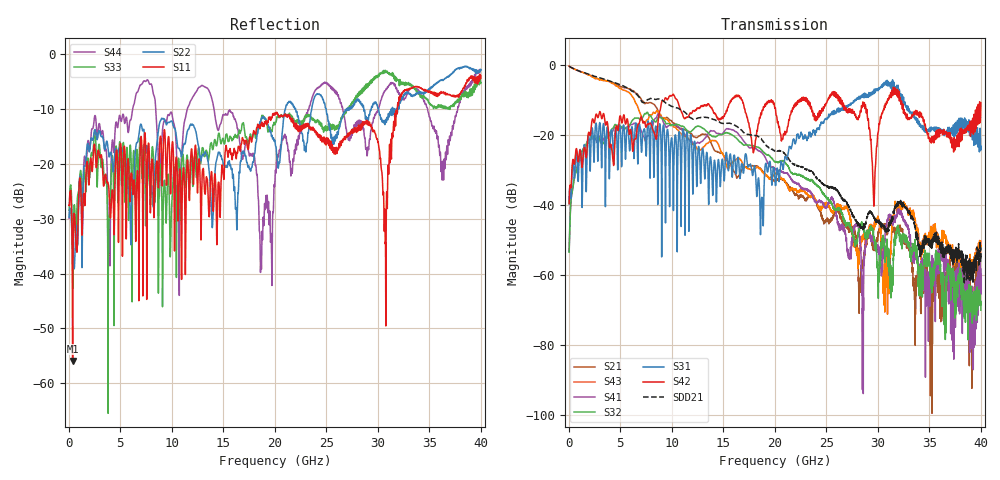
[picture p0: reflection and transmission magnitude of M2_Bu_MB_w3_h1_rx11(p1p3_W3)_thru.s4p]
! S11 = S11
! S12 = S12
! S13 = S13
! S14 = S14
! S21 = S21
! S22 = S22
! S23 = S23
! S24 = S24
! S31 = S31
! S32 = S32
! S33 = S33
! S34 = S34
! S41 = S41
! S42 = S42
! S43 = S43
! S44 = S44
! FILE: \\englab.brocade.com\shares\Groups\SIT\Work\Shaohua\IEEE_channels\M2_Bu_MB_w3_h1_rx11(p1p3_W3)_thru.s4p
!$DUT_CFG_DESC: Default 4-Port Configuration
!$NUMBER_PORTS: 4
!$DIFF_PORT_MAP: 1|2P|2|2P|0|UC|0|UC|
!$PORT_MAP: PNA 1|1|<<<<<<|TS 2|2|>>>>>>|PNA 2|3|<<<<<<|TS 4|4|>>>>>>|
# MHz S RI R 50.00
! FREQ  S11  S12  S13  S14
!  S21  S22  S23  S24
!  S31  S32  S33  S34
!  S41  S42  S43  S44
!  REAL  IMAG  REAL  IMAG  REAL  IMAG  REAL  IMAG
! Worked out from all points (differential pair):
!   3996 points, 50 MHz to 40 GHz, reference 50 ohm
!   strongest paths, dB at 50 MHz, 10.04 GHz, 20.03 GHz, 30.02 GHz, 40 GHz:
!     S42: -39.7, -8.7, -12.3, -19.3, -10.8
!     S31: -39.6, -21.7, -33.3, -7.2, -23.2
!     S32: -53.5, -17.1, -27.7, -61.3, -70.1
!     S41: -53.4, -17.2, -29.7, -53.3, -58.3
!     S43: -0.4, -17.1, -31.1, -43.7, -50.4
!     S21: -0.3, -16.3, -32.9, -48.9, -60.1
!   taken as a pair (ports 3,1 in; 4,2 out), SDD21 dB: -0.4, -11.9, -24.5, -44.9, -52.1
!   lowest |S11| = -55.9 dB at 390 MHz (marker M1), VSWR 1.00, Z = 50.1 - j0.151 ohm
!   |S11| at or under -10 dB: start of sweep to 31.89 GHz
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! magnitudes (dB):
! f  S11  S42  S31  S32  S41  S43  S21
! 50 MHz  -27.5  -39.7  -39.6  -53.5  -53.4  -0.4  -0.3
! 390 MHz  -55.9  -27.4  -28.2  -35.5  -35.6  -0.9  -0.9
! 15.45 GHz  -18.6  -12.1  -29.3  -19.4  -18.2  -29.7  -27.6
! 18.67 GHz  -13.0  -13.7  -41.5  -24.1  -24.8  -29.8  -29.8
! 29.62 GHz  -14.1  -40.4  -8.1  -50.2  -49.9  -47.1  -52.9
! 30.74 GHz  -34.6  -11.0  -4.9  -52.5  -47.5  -55.9  -47.1
! 40 GHz  -4.0  -10.8  -23.2  -70.1  -58.3  -50.4  -60.1
